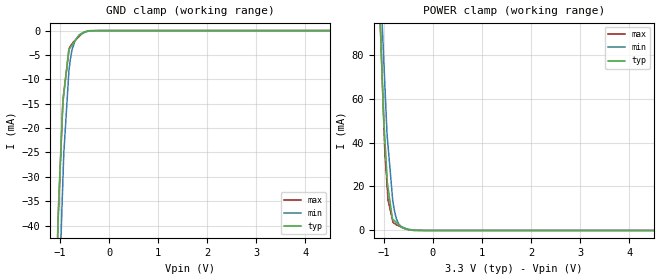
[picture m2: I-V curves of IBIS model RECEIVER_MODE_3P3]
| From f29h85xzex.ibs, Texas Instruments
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|   Model Cell RECEIVER_MODE_3P3
|RECEIVER_MODE_3P3
[Model]   RECEIVER_MODE_3P3
Model_type   Input
Polarity   Non-Inverting
Vinl = 0.8
Vinh = 2
|   typ   min   max
C_comp   0.36pF   0.33pF   0.38pF
[Model Spec]
Vinl   0.8   0.8   0.8
Vinh   2   2   2
[Temperature Range]   25   155   -40
[Voltage Range]   3.3   2.8   3.63
| Nom Voltages:
|   BIASFET=3.3, VDD=1.23, VDDS=3.3, VSS=0
| Min Voltages:
|   BIASFET=2.97, VDD=1.08, VDDS=2.8, VSS=0
| Max Voltages:
|   BIASFET=3.63, VDD=1.32, VDDS=3.63, VSS=0
[Power Clamp Reference]   3.3   2.8   3.63
[GND Clamp Reference]   0   0   0
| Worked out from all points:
|   GND clamp passes 1 mA (typ) near -0.62 V on its own axis
|   POWER clamp passes 1 mA (typ) near -0.60 V on its own axis
[GND Clamp]
|   Voltage   I(typ)   I(min)   I(max)
-3.3V     -1.461A    -1.198A    -2.144A
-1.047V   -41.8mA    -64.08mA   -40.47mA
-1.024V   -33.93mA   -55.24mA   -34.8mA
-945.8mV  -15.13mA   -31.55mA   -15.38mA
-940mV    -14.6mA    -29.81mA   -13.95mA
-925.1mV  -13.23mA   -25.31mA   -12.74mA
-824.5mV  -3.967mA   -9.041mA   -4.536mA
-813.6mV  -3.808mA   -7.742mA   -3.648mA
-758mV    -2.999mA   -4.06mA    -2.748mA
-702.3mV  -2.19mA    -2.274mA   -2.099mA
-523.4mV  -335.2uA   -471.9uA   -461.1uA
6.6V      0A         0A         0A
[POWER Clamp]
|   Voltage   I(typ)   I(min)   I(max)
-3.3V     1.933A     2.239A     2.093A
-1.07V    91.49mA    120.7mA    92.39mA
-1.035V   70.36mA    95.86mA    70.59mA
-1.024V   63.26mA    88.7mA     63.26mA
-978.5mV  41.35mA    65.87mA    35.48mA
-934.3mV  24.19mA    43.64mA    20.41mA
-915.1mV  19.57mA    38.64mA    13.84mA
-824.5mV  5.227mA    15.16mA    4.779mA
-795.8mV  4.659mA    10.44mA    3.397mA
-731.3mV  3.387mA    4.549mA    2.458mA
-616.2mV  1.118mA    1.462mA    1.27mA
6.6V      0A         0A         0A
